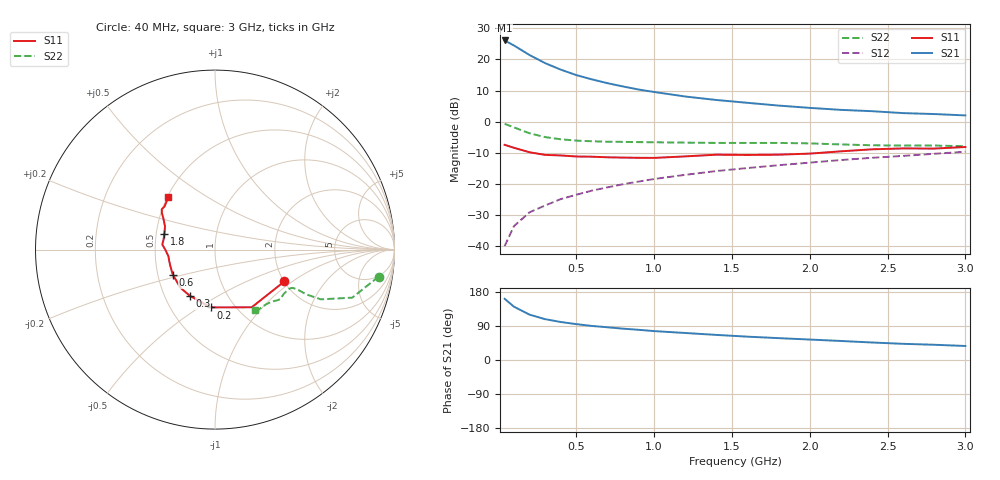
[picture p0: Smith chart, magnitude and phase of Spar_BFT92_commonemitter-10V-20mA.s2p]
! Filename:  BFT92J.S2P  Version:  2.0
! NXP part #: BFT92  Date: May 1990
! Bias condition: Vce=-10V, Ic=-20mA
#  MHz  S  MA  R  50
! Freq  S11  S21  S12  S22  !GUM [dB]
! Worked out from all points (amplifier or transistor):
!   21 points, 40 MHz to 3 GHz, reference 50 ohm
!   highest |S21| = 26.1 dB at 40 MHz (marker M1)
!   |S21| within 3 dB of that: start of sweep to 145.2 MHz
!   unconditionally stable (mu >= 1): 543.4 MHz to 2.264 GHz
!   at 300 MHz: K = 0.86, MSG = 22.9 dB, |S12| = -26.9 dB
!   at 1 GHz: K = 1.07, MAG = 12.4 dB, |S12| = -18.4 dB
!   at 3 GHz: K = 0.92, MSG = 5.8 dB, |S12| = -9.7 dB
!   S11 on the Smith chart (normalised r, x): 40 MHz: 2.01, -0.87; 200 MHz: 0.78, -0.56; 300 MHz: 0.67, -0.38; 600 MHz: 0.60, -0.18; 1.8 GHz: 0.55, +0.10; 3 GHz: 0.51, +0.35
40  0.425 -24.7  20.2 161.5  0.01 81.3  0.924 -9.4
100  0.381 -57.5  16.76 140.7  0.021 72.4  0.81 -19.3
200  0.323 -94.3  11.79 119.7  0.035 68.0  0.651 -25.2
300  0.293 -118.5  8.733 107.8  0.045 68.2  0.566 -26.1
400  0.287 -132.3  6.869 100.3  0.057 69.4  0.522 -25.9
500  0.276 -141.6  5.614 94.7  0.067 70.5  0.497 -26.0
600  0.274 -148.8  4.791 89.9  0.078 71.1  0.485 -26.2
700  0.268 -154.7  4.163 86.4  0.088 71.7  0.477 -26.6
800  0.265 -159.8  3.681 82.7  0.099 72.1  0.474 -27.1
900  0.263 -166.2  3.29 79.7  0.109 72.0  0.47 -27.5
1000  0.262 -171.7  3.002 76.3  0.12 72.1  0.467 -28.2
1200  0.277 -179.9  2.54 71.3  0.14 71.9  0.461 -30.1
1400  0.295 174.5  2.232 66.2  0.161 71.6  0.456 -32.5
1600  0.292 169.4  2.011 61.6  0.18 71.0  0.456 -35.1
1800  0.295 163.0  1.815 57.7  0.2 70.8  0.456 -37.2
2000  0.307 155.1  1.667 54.0  0.22 70.4  0.448 -39.1
2200  0.334 149.2  1.549 50.2  0.242 69.9  0.431 -42.1
2400  0.36 145.3  1.475 46.2  0.263 69.1  0.418 -46.5
2600  0.372 142.9  1.374 42.7  0.282 68.3  0.413 -51.2
2800  0.37 139.3  1.327 40.2  0.305 68.0  0.414 -54.2
3000  0.392 131.6  1.261 37.0  0.329 66.9  0.403 -56.7
